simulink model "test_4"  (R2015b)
settings: Solver=VariableStepAuto  StartTime=0.0  StopTime=1  RelTol=1e-3
undefined symbols (not defined in the file or in its folder): fir1
libraries: dsparch4 x1

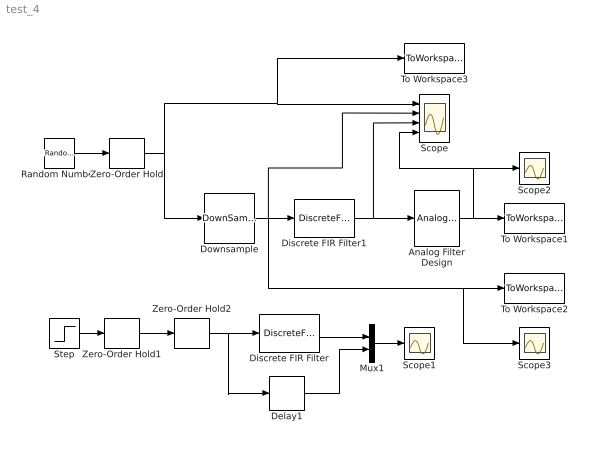
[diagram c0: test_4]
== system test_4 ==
  Analog Filter Design : dsparch4/Analog Filter Design  method=Butterworth  filttype=Lowpass  N=8  Wlo=2*pi*10  Whi=80  Rp=2  Rs=40
  Delay1 : Delay  DelayLength=8
  Discrete FIR Filter : DiscreteFir  Coefficients=fir1(16,0.005)
  Discrete FIR Filter1 : DiscreteFir  Coefficients=fir1(16,0.5)
  Downsample : DownSample  N=4  RateOptions=Allow multirate processing
  Mux1 : Mux  Inputs=2
  Random Number : RandomNumber  SampleTime=0
  Scope : Scope  NumInputPorts=4
  Scope1 : Scope
  Scope2 : Scope
  Scope3 : Scope
  Step : Step  Time=0.2  SampleTime=0
  To Workspace1 : ToWorkspace  VariableName=y2  SaveFormat=Structure With Time  SampleTime=-1
  To Workspace2 : ToWorkspace  VariableName=y3  SaveFormat=Timeseries  SampleTime=-1
  To Workspace3 : ToWorkspace  VariableName=y1  SaveFormat=Timeseries  SampleTime=-1
  Zero-Order Hold : ZeroOrderHold  SampleTime=0.01
  Zero-Order Hold1 : ZeroOrderHold  SampleTime=0.01
  Zero-Order Hold2 : ZeroOrderHold  SampleTime=0.005
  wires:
  Random Number/1 -> Zero-Order Hold/1
  Zero-Order Hold/1 -> Scope/1, To Workspace3/1, Downsample/1
  Discrete FIR Filter/1 -> Mux1/1
  Mux1/1 -> Scope1/1
  Step/1 -> Zero-Order Hold1/1
  Delay1/1 -> Mux1/2
  Discrete FIR Filter1/1 -> Scope/3, Analog Filter Design/1
  Zero-Order Hold1/1 -> Zero-Order Hold2/1
  Analog Filter Design/1 -> Scope2/1, Scope/4, To Workspace1/1
  Downsample/1 -> Scope/2, Scope3/1, To Workspace2/1, Discrete FIR Filter1/1
  Zero-Order Hold2/1 -> Delay1/1, Discrete FIR Filter/1
